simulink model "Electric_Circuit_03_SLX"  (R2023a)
settings: Solver=ode23s  StartTime=0.0  StopTime=10.0  MaxStep=0.001  RelTol=1e-3
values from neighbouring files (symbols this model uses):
  C_3 = 0.001*F    (= 0.001)    [Electric_Circuit_03_EQN.m]    (also in Electric_Circuit_03_SLX_m.m; BIG_EC_Simscape_EQN.m; BIG_EC_Simscape_SLX_m.m; Electric_Circuit_07_EQN.m)
  C_6 = 0.001*F    (= 0.001)    [Electric_Circuit_03_EQN.m]    (also in Electric_Circuit_03_SLX_m.m; Electric_Circuit_01_EQN.m; Electric_Circuit_01_SLX_m.m; Electric_Circuit_06_EQN.m)
  I_2_0 = 0*A    (= 0)    [Electric_Circuit_03_SLX_m.m]    (also in Electric_Circuit_02_SLX_m.m; Electric_Circuit_06_SLX_m.m; Electric_Circuit_08_SLX_m.m; Electric_Circuit_09_SLX_m.m)
  I_4_0 = 0*A    (= 0)    [Electric_Circuit_03_SLX_m.m]    (also in Electric_Circuit_02_SLX_m.m; Electric_Circuit_04_SLX_m.m; Electric_Circuit_05_SLX_m.m; Electric_Circuit_07_SLX_m.m)
  L_2 = 0.002*H    (= 0.002)    [Electric_Circuit_03_EQN.m]    (also in Electric_Circuit_03_SLX_m.m; Electric_Circuit_02_EQN.m; Electric_Circuit_02_SLX_m.m; Electric_Circuit_06_EQN.m)
  L_4 = 0.002*H    (= 0.002)    [Electric_Circuit_03_EQN.m]    (also in Electric_Circuit_03_SLX_m.m; Electric_Circuit_02_EQN.m; Electric_Circuit_02_SLX_m.m; Electric_Circuit_04_EQN.m)
  R_5 = 100*Ohm    (= 100)    [Electric_Circuit_03_EQN.m]    (also in Electric_Circuit_03_SLX_m.m; Electric_Circuit_07_EQN.m; Electric_Circuit_07_SLX_m.m; Inductive_Circuit_1_EQN.m)
  R_7 = 100*Ohm    (= 100)    [Electric_Circuit_03_EQN.m]    (also in Electric_Circuit_03_SLX_m.m; BIG_EC_Simscape_EQN.m; BIG_EC_Simscape_SLX_m.m; Electric_Circuit_06_EQN.m)
  Ts = Tfin/Nr_Ts_Points    (= 0.0006)    [Electric_Circuit_03_SLX_m.m]    (also in BIG_EC_Simscape_SLX_m.m = 0.0003; Car_Dumper_SLX_m.m = 0.0022779; Electric_Circuit_01_SLX_m.m = 0.005; Electric_Circuit_02_SLX_m.m = 0.000480145)
  V_1_0 = 10*V    (= 10)    [Electric_Circuit_03_SLX_m.m]    (also in BIG_EC_Simscape_SLX_m.m; Electric_Circuit_02_SLX_m.m; Electric_Circuit_04_SLX_m.m; Electric_Circuit_05_SLX_m.m)
  V_3_0 = 0*V    (= 0)    [Electric_Circuit_03_SLX_m.m]    (also in BIG_EC_Simscape_SLX_m.m; Electric_Circuit_07_SLX_m.m; Electric_Circuit_11_SLX_m.m; Electrical_Transformer_SLX_m.m)
  V_6_0 = 0*V    (= 0)    [Electric_Circuit_03_SLX_m.m]    (also in Electric_Circuit_01_SLX_m.m; Electric_Circuit_06_SLX_m.m; Electric_Circuit_08_SLX_m.m; Electric_Circuit_10_SLX_m.m)
  V_8_0 = 0*V    (= 0)    [Electric_Circuit_03_SLX_m.m]    (also in BIG_EC_Simscape_SLX_m.m; Electric_Circuit_04_SLX_m.m; Electric_Circuit_09_SLX_m.m; Electric_Circuit_11_SLX_m.m)

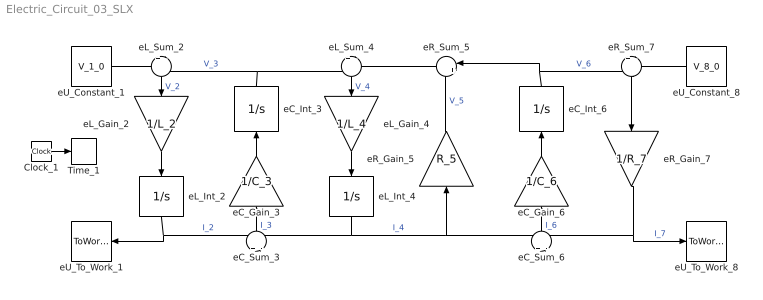
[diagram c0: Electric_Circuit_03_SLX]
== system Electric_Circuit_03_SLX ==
  Clock_1 : Clock
  Time_1 : ToWorkspace  VariableName=t  SaveFormat=Timeseries  SampleTime=Ts
  eC_Gain_3 : Gain  Gain=1/C_3  Multiplication=Matrix(K*u)
  eC_Gain_6 : Gain  Gain=1/C_6  Multiplication=Matrix(K*u)
  eC_Int_3 : Integrator  InitialCondition=V_3_0
  eC_Int_6 : Integrator  InitialCondition=V_6_0
  eC_Sum_3 : Sum  Inputs=+|-
  eC_Sum_6 : Sum  Inputs=+|-
  eL_Gain_2 : Gain  Gain=1/L_2  Multiplication=Matrix(K*u)
  eL_Gain_4 : Gain  Gain=1/L_4  Multiplication=Matrix(K*u)
  eL_Int_2 : Integrator  InitialCondition=I_2_0
  eL_Int_4 : Integrator  InitialCondition=I_4_0
  eL_Sum_2 : Sum  Inputs=+|-
  eL_Sum_4 : Sum  Inputs=+|-
  eR_Gain_5 : Gain  Gain=R_5  Multiplication=Matrix(K*u)
  eR_Gain_7 : Gain  Gain=1/R_7  Multiplication=Matrix(K*u)
  eR_Sum_5 : Sum  Inputs=|++
  eR_Sum_7 : Sum  Inputs=+|-
  eU_Constant_1 : Constant  Value=V_1_0
  eU_Constant_8 : Constant  Value=V_8_0
  eU_To_Work_1 : ToWorkspace  VariableName=I_1_0  SaveFormat=Timeseries  SampleTime=Ts
  eU_To_Work_8 : ToWorkspace  VariableName=I_8_0  SaveFormat=Timeseries  SampleTime=Ts
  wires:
  eU_Constant_1/1 -> eL_Sum_2/1
  eC_Int_3/1 -> eL_Sum_2/2, eL_Sum_4/1  "V_3"
  eL_Int_2/1 -> eU_To_Work_1/1, eC_Sum_3/1  "I_2"
  eL_Sum_2/1 -> eL_Gain_2/1  "V_2"
  eL_Gain_2/1 -> eL_Int_2/1
  eL_Int_4/1 -> eC_Sum_3/2, eR_Gain_5/1, eC_Sum_6/1  "I_4"
  eC_Sum_3/1 -> eC_Gain_3/1  "I_3"
  eC_Gain_3/1 -> eC_Int_3/1
  eR_Sum_5/1 -> eL_Sum_4/2
  eL_Sum_4/1 -> eL_Gain_4/1  "V_4"
  eL_Gain_4/1 -> eL_Int_4/1
  eC_Int_6/1 -> eR_Sum_5/1, eR_Sum_7/1  "V_6"
  eR_Gain_5/1 -> eR_Sum_5/2  "V_5"
  eR_Gain_7/1 -> eC_Sum_6/2, eU_To_Work_8/1  "I_7"
  eC_Sum_6/1 -> eC_Gain_6/1  "I_6"
  eC_Gain_6/1 -> eC_Int_6/1
  eU_Constant_8/1 -> eR_Sum_7/2
  eR_Sum_7/1 -> eR_Gain_7/1
  Clock_1/1 -> Time_1/1
